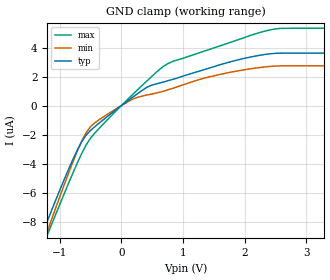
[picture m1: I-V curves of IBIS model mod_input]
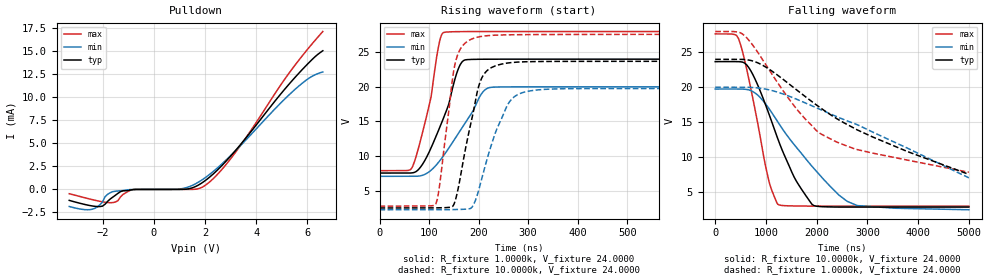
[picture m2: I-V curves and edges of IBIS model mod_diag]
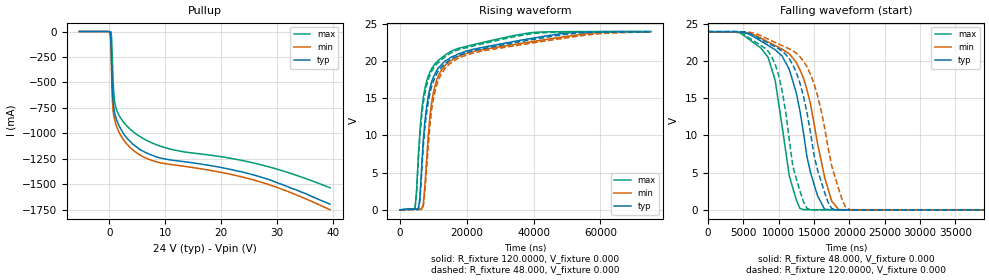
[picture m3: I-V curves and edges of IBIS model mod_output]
| IBIS (I/O, Buffer, Information, Specification) Model, officially
| electronic behavioral standard for Buffer structures of digital pins.
[IBIS ver]  4.0
[File name] vni2140j_ibis.ibs
[File Rev]  1.0
[Date]   16 Feb 2024
[Source]   CAD & Design Services (Catania) - STMicroelectronics
[Notes]
   (Note1)  This IBIS model includes PowerSSO-12 ceramic package data
   (Note2)  This IBIS model has some Notes about the non-monotonicity
   of the I-V curves, but they are not indicative of problems
   inside the model;
[Disclaimer]
   Customers are solely responsible for all aspects of their
   own product designs or applications using this IBIS Model.
   STMicroelectronics assumes no liability for Custmer Designs
   and applications associated to this IBIS Model.
   In the use of this IBIS Model Customer shall not modify,
   disassemble, alter this Model in whole or in part.
   If Customers do not accept these terms, the IBIS Model
   may not be used. For any problems or modifications please
   contact STMicroelectronics (www.st.com).
[Copyright] (c) 2024 STMicroelectronics
|   Component VNI2140J
[Component] VNI2140J
[Manufacturer] STMicroelectronics
[Package]
| variable  typ   min   max
R_pkg   0.0   0.0   0.0
L_pkg   0.0H   0.0H   0.0H
C_pkg   0.0F   0.0F   0.0F
[Pin]   signal_name   model_name   R_pin   L_pin   C_pin
1   NC   NC   0.0   0.0   0.0
2   INP1   mod_input   25.151m   1.8569nH   0.2710pF
3   DIAG1   mod_diag   26.615m   1.9638nH   0.2818pF
4   GND   GND   21.397m   1.6902nH   0.2631pF
5   DIAG1   mod_diag   20.931m   1.6859nH   0.2587pF
6   INP2   mod_input   20.976m   1.6983nH   0.2385pF
7   VCC   POWER   0.5754m   1.2255nH   0.5276pF
8   OUT1   mod_output   26.132m   1.9519nH   0.2653pF
9   OUT1   mod_output   12.598m   1.5412nH   0.3347pF
10   OUT2   mod_output   12.573m   1.5393nH   0.3335pF
11   OUT2   mod_output   25.920m   1.9601nH   0.2651pF
12   VCC   POWER   0.5755m   1.2269nH   0.5276pF
13   EXPVCC   POWER   0.0033m   0.0431nH   0.5276pF
| Models and submodels in the file (3): mod_input (Input), mod_diag (Open_drain), mod_output (Open_source)
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|   Model mod_input
[Model]   mod_input
Model_type Input
Vinl   =   0.800V
Vinh   =   2.200V
C_comp   8.056pF   7.690pF   8.820pF
[Temperature Range]  25.0000   85.0000   -40.0000
[Voltage Range]   3.3000V   3.0000V   3.6000V
[GND_clamp]
|Voltage   I(typ)   I(min)   I(max)
-3.3V     -32.56uA   -34.48uA   -31.48uA
-1.34V    -9.492uA   -10.35uA   -10.4uA
-1.27V    -8.728uA   -9.511uA   -9.666uA
-1.2V     -7.971uA   -8.675uA   -8.929uA
-780mV    -3.671uA   -3.842uA   -4.611uA
-570mV    -2.033uA   -1.867uA   -2.714uA
-430mV    -1.453uA   -1.186uA   -1.893uA
-10mV     -31.46nA   -24.94nA   -41.98nA
410mV     1.257uA    730.4nA    1.682uA
830mV     1.802uA    1.189uA    3.045uA
2.37V     3.551uA    2.685uA    5.18uA
3.28V     3.62uA     2.744uA    5.335uA
|   Model mod_diag
[Model]   mod_diag
Model_type Open_drain
Polarity   Non-Inverting
Enable   Active-Low
Vmeas  =   12.00V
Vref   =   24.00V
Cref   =   50.0pF
Rref   =   10k
C_comp   8.056pF   7.690pF   8.820pF
[Temperature Range]  25.0000   85.0000   -40.0000
[Voltage Range]   3.3000V   3.0000V   3.6000V
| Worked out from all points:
|   rising waveform, R_fixture 1.0000k, V_fixture 24.0000: 20-80 % time 48.8ns typ, 69.2ns min, 33.1ns max; typ from 7.54 V to 24 V
|   rising waveform, R_fixture 10.0000k, V_fixture 24.0000: 20-80 % time 35.3ns typ, 48.6ns min, 25.8ns max; typ from 2.5 V to 23.7 V
|   falling waveform, R_fixture 10.0000k, V_fixture 24.0000: 20-80 % time 682ns typ, 1.13us min, 400ns max; typ from 23.6 V to 2.81 V
|   falling waveform, R_fixture 1.0000k, V_fixture 24.0000: 20-80 % time 2.37us typ, 2.38us min, 1.56us max; typ from 24 V to 7.5 V
[Pulldown]
|Voltage   I(typ)   I(min)   I(max)
-3.3V     -1.189mA   -1.852mA   -466uA
-2.4V     -1.795mA   -2.148mA   -1.106mA
-2V       -1.812mA   -1.365mA   -1.347mA
-1.9V     -1.601mA   -789uA     -1.392mA
-1.6V     -841.1uA   -244.3uA   -1.43mA
-1.3V     -241.9uA   -149.5uA   -820.9uA
-800mV    -18.17uA   -9.868uA   -14.23uA
1.1V      2.838uA    80.7uA     0A
2V        934.4uA    1.253mA    421.8uA
3.2V      4.244mA    4.216mA    4.051mA
5.5V      12.09mA    10.8mA     13.41mA
6.6V      15.03mA    12.73mA    17.11mA
[Ramp]
| variable   typ   min   max
dV/dt_r   0.1179/14.9399n   96.8400m/19.7987n  0.1403/11.1259n
dV/dt_f   6.9600m/0.1176u   1.0800m/0.1424u   45.5400m/0.1647u
R_load = 50.0000
[Rising Waveform]
R_fixture= 1.0000k
V_fixture= 24.0000
V_fixture_min= 20.0000
V_fixture_max= 28.0000
|time   V(typ)   V(min)   V(max)
0s        7.542V     7.064V     7.884V
65.6ns    7.562V     7.064V     8.303V
81.6ns    8.289V     7.122V     11.93V
100.8ns   10.67V     7.76V      17.49V
120ns     13.85V     9.166V     26.12V
129.6ns   15.55V     10.08V     27.81V
166.4ns   23.55V     14.05V     27.94V
204.8ns   23.95V     18.86V     27.95V
222.4ns   23.96V     19.87V     27.95V
800ns     23.96V     19.97V     27.94V
[Rising Waveform]
R_fixture= 10.0000k
V_fixture= 24.0000
V_fixture_min= 20.0000
V_fixture_max= 28.0000
|time   V(typ)   V(min)   V(max)
0s        2.502V     2.245V     2.769V
113.6ns   2.517V     2.25V      3.039V
121.6ns   2.526V     2.252V     5.933V
152ns     3.359V     2.274V     23.14V
185.6ns   15.06V     2.541V     26.85V
200ns     20.01V     5.024V     27.17V
214.4ns   22.11V     8.869V     27.33V
256ns     23.38V     17.02V     27.47V
284.8ns   23.56V     19.04V     27.5V
800ns     23.66V     19.73V     27.54V
[Falling Waveform]
R_fixture= 10.0000k
V_fixture= 24.0000
V_fixture_min= 20.0000
V_fixture_max= 28.0000
|time   V(typ)   V(min)   V(max)
0s        23.64V     19.71V     27.6V
461.6ns   23.63V     19.71V     26.9V
741.6ns   21.79V     19.35V     18.36V
1.051us   16.3V      17.01V     6.769V
1.232us   12.63V     15.03V     3.221V
1.592us   6.629V     11.44V     2.971V
1.952us   3.008V     8.291V     2.949V
2.44us    2.814V     4.525V     2.937V
2.8us     2.814V     3.029V     2.937V
5us       2.814V     2.429V     2.937V
[Falling Waveform]
R_fixture= 1.0000k
V_fixture= 24.0000
V_fixture_min= 20.0000
V_fixture_max= 28.0000
|time   V(typ)   V(min)   V(max)
0s        23.96V     19.97V     27.95V
467.6ns   23.96V     19.97V     27.86V
579.6ns   23.94V     19.97V     27.35V
960.4ns   23.01V     19.75V     23.62V
1.565us   19.82V     18.37V     17.23V
1.985us   17.49V     17.05V     13.83V
2.097us   16.9V      16.69V     13.23V
2.8us     13.86V     14.61V     11.04V
3.8us     10.73V     11.21V     9.522V
5us       7.5V       7V         7.8V
|   Model mod_output
[Model]   mod_output
Model_type Open_source
Polarity   Non-Inverting
Enable   Active-Low
Vmeas  =   1.650V
Vref   =   0.0V
Cref   =   50.0pF
Rref   =   100
C_comp   125.50pF   123.60pF   128.40pF
[Temperature Range]  25.0000   85.0000   -40.0000
[Voltage Range]   24.000V   24.000V   24.200V
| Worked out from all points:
|   slope of the pullup table from 0 to 3.6 V, typ, clamps not added: 3.36 ohm
|   rising waveform, R_fixture 120.0000, V_fixture 0.000: 20-80 % time 5.31us typ, 5.38us min, 4.55us max; typ from 0 V to 24 V
|   rising waveform, R_fixture 48.000, V_fixture 0.000: 20-80 % time 5.92us typ, 5.82us min, 4.96us max; typ from 0 V to 23.9 V
|   falling waveform, R_fixture 48.000, V_fixture 0.000: 20-80 % time 3.22us typ, 3.55us min, 2.53us max; typ from 23.9 V to 0 V
|   falling waveform, R_fixture 120.0000, V_fixture 0.000: 20-80 % time 3.52us typ, 3.82us min, 2.68us max; typ from 24 V to 0 V
[Pullup]
|Voltage   I(typ)   I(min)   I(max)
-5.4V     169.5uA    171.4uA    177.3uA
0V        -787.6uA   -7.242mA   20.71uA
200mV     -46.99mA   -78.09mA   -1.272mA
300mV     -152.6mA   -222.9mA   -6.682mA
500mV     -548.8mA   -646.2mA   -246.8mA
700mV     -704.3mA   -799.1mA   -536.4mA
900mV     -787.1mA   -860mA     -680.2mA
2.1V      -963.5mA   -1.027A    -857.4mA
4.7V      -1.128A    -1.184A    -1.003A
10.7V     -1.259A    -1.304A    -1.151A
26.9V     -1.425A    -1.475A    -1.305A
39.5V     -1.696A    -1.75A     -1.534A
[Ramp]
| variable   typ   min   max
dV/dt_r   17.270/15.67u   17.180/15.35u   17.290/15.45u
dV/dt_f   15.960/4.276u   15.930/4.126u   15.990/4.282u
R_load = 50.0000
[Rising Waveform]
R_fixture= 120.0000
V_fixture= 0.000
V_fixture_min= 0.000
V_fixture_max= 0.000
|time   V(typ)   V(min)   V(max)
0s        569.2nV    1.194uV    581nV
4.5us     88.09mV    85.6mV     85.97mV
6us       1.66V      65.71mV    10.65V
7us       9.336V     738.9mV    15.11V
8us       13.86V     6.721V     17.3V
9.5us     17.23V     14.44V     18.98V
11us      18.72V     17.44V     19.88V
14us      20.13V     19.63V     20.96V
39us      23.01V     22.56V     23.81V
75us      23.97V     23.95V     23.98V
[Rising Waveform]
R_fixture= 48.000
V_fixture= 0.000
V_fixture_min= 0.000
V_fixture_max= 0.000
|time   V(typ)   V(min)   V(max)
0s        227.8nV    477.8nV    232.5nV
4.5us     35.26mV    34.26mV    34.86mV
5us       32.7mV     32.69mV    2.277V
6us       1.207V     26.27mV    9.96V
7us       8.579V     431.5mV    14.38V
8.5us     14.55V     8.684V     17.52V
10us      17.26V     14.91V     19V
14us      19.84V     19.26V     20.73V
39.5us    22.87V     22.44V     23.69V
75us      23.92V     23.89V     23.95V
[Falling Waveform]
R_fixture= 48.000
V_fixture= 0.000
V_fixture_min= 0.000
V_fixture_max= 0.000
|time   V(typ)   V(min)   V(max)
0s        23.92V     23.88V     23.95V
4.5us     23.9V      23.87V     23.8V
8.5us     22.11V     22.58V     20.51V
9.5us     21.54V     22.08V     17.44V
11.5us    18.89V     20.99V     4.567V
13us      13.34V     18.83V     195.5mV
15.5us    1.885V     8.908V     488.7uV
17.5us    2.081mV    1.165V     198.9uV
18.5us    726.7uV    16.63mV    122.6uV
60us      18.86uV    11.08uV    31.36uV
[Falling Waveform]
R_fixture= 120.0000
V_fixture= 0.000
V_fixture_min= 0.000
V_fixture_max= 0.000
|time   V(typ)   V(min)   V(max)
0s        23.97V     23.95V     23.98V
4.5us     23.96V     23.95V     23.89V
9us       22.17V     22.73V     20.64V
10.5us    21.33V     22.07V     15.97V
12us      19.51V     21.39V     5.868V
14us      13.09V     19.21V     179.2mV
15.5us    5.326V     15.34V     2.055mV
17us      975mV      8.297V     901.2uV
20us      1.336mV    35.01mV    301.9uV
60us      34.69uV    30.41uV    77.29uV
